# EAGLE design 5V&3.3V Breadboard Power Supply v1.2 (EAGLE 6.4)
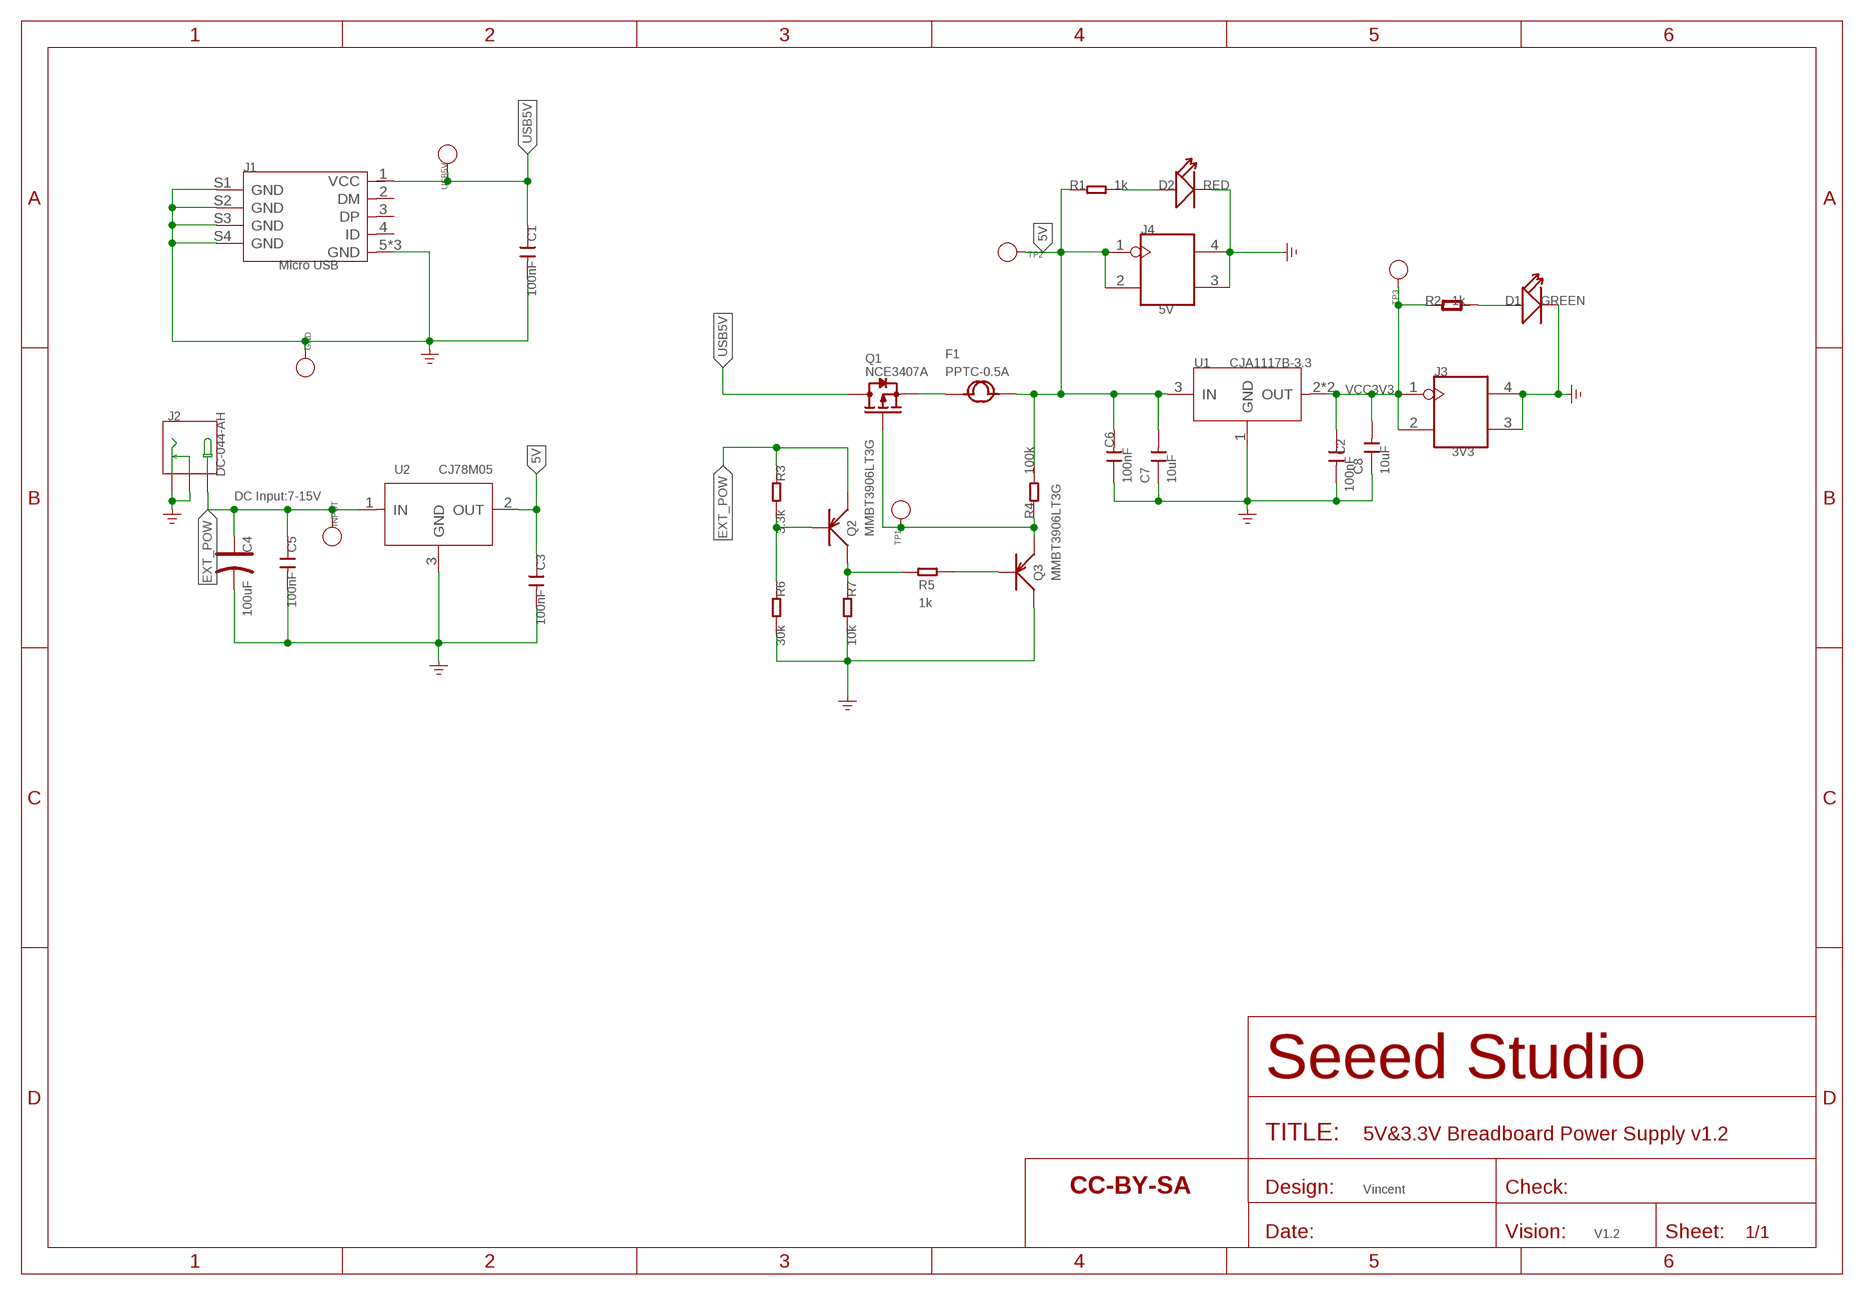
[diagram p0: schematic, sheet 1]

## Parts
C1  100nF  CAP-0603  [C0603]
C2  100nF  CAP-0603  [C0603]
C3  100nF  CAP-0603  [C0603]
C4  100uF  CAP_ELECTRO_D  [ELECTRO-SMD-D]
C5  100nF  CAP-0603  [C0603]
C6  100nF  CAP-0603  [C0603]
C7  10uF  CAP-0805  [C0805]
C8  10uF  CAP-0805  [C0805]
D1  GREEN  LED-0603  [LED-0603]
D2  RED  LED-0603  [D0603]
F1  PPTC-0.5A  FUSE'1206'  [F1206]
GND  DNP  PAD-TEST-POINT'4545'  [TP_4545]
INPUT  DNP  PAD-TEST-POINT'4545'  [TP_4545]
J1  Micro USB  USB-MICRO-5P'5+4P'  [5+4P-SMD-0.65-B]
J2  DC-044-AH  POWER-JACK-DC'DC-044'  [3P-L11.6*W9.6*H7.0MM]
J3  3V3  HEADER-2X2P-2.54  [2X2P-2.54-65/35MIL]
J4  5V  HEADER-2X2P-2.54  [2X2P-2.54-65/35MIL]
Q1  NCE3407A  MOSFET-P'SI2323CDS/SI2305DS<BR>'  [SOT23]
Q2  MMBT3906LT3G  TRANSISTOR-PNP-SOT23  [SOT23]
Q3  MMBT3906LT3G  TRANSISTOR-PNP-SOT23  [SOT23]
R1  1k  R-0603  [R0603]
R2  1k  R-0603  [R0603]
R3  3.3k  R-0603  [R0603]
R4  100k  R-0603  [R0603]
R5  1k  R-0603  [R0603]
R6  30k  R-0603  [R0603]
R7  10k  R-0603  [R0603]
TP1  DNP  PAD-TEST-POINT'4545'  [TP_4545]
TP2  DNP  PAD-TEST-POINT'4545'  [TP_4545]
TP3  DNP  PAD-TEST-POINT'4545'  [TP_4545]
U1  CJA1117B-3.3  PMIC-CJ1117'SOT89'  [SOT-89]
U2  CJ78M05  PMIC-CJ78M05CJ  [TO-252]
U$3  SEEEDSTUDIO-OPEN-SCH-FRAME  [SEEEDSTUDIO-PCB-FRAME]
USB5V  DNP  PAD-TEST-POINT'4545'  [TP_4545]

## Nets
5V: C3.1 C6.2 C7.2 F1.2 J4.1 J4.2 R1.1 R4.2 TP2.T U1.3(IN) U2.2(OUT)
EXT_POW: C4.+ C5.1 INPUT.T J2.+ Q2.2(E) R3.1 U2.1(IN)
EXT_PWR_SIG: Q1.1(G) Q3.2(E) R4.1 TP1.T
GND: C1.2 C2.2 C3.2 C4.- C5.2 C6.1 C7.1 C8.1 D1.- D2.- GND.T J1.5(GND) J1.S1(GND) J1.S2(GND) J1.S3(GND) J1.S4(GND) J1.S5(GND) J1.S6(GND) J2.- J2.CDN J3.3 J3.4 J4.3 J4.4 Q3.3(C) R6.2 R7.2 U1.1(GND) U2.3(GND) ; supply symbol labelled GND_POWER
N$1: D1.+ R2.2
N$2: Q2.1(B) R3.2 R6.1
N$3: D2.+ R1.2
N$8: Q3.1(B) R5.2
N$9: Q2.3(C) R5.1 R7.1
P5V [usbvcc]: F1.1 Q1.2(S)
USB5V: C1.1 J1.1(VCC) Q1.3(D) USB5V.T
VCC3V3: C2.1 C8.2 J3.1 J3.2 R2.1 TP3.T U1.2(OUT) U1.4(OUT)
Unconnected: J1.2(DM) J1.3(DP) J1.4(ID)

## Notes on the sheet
- DC Input:7-15V
- Vincent
- V1.2

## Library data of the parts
C1-C3 C5-C8 = OPL:CAP: Ceramic Capacitors
C4 = Discrete:CAP*: Electrolytic Capacitors,Tantalum Capacitors and Super Capacitors
D1 = OPL:LED
D2 = Discrete:LED*
F1 = Discrete:FUSE
GND INPUT TP1-TP3 USB5V = Discrete:PAD-TEST-POINT; PARTNO: DNP
J1 = Connector-new:USB-MICRO-5P: 5+4P-SMD-0.65-B:320010000;5+2P-SMD-0.65-AB:340032001
J2 = Connector-new:POWER-JACK-DC: 3P-L11.6*W9.6*H7.0MM:320120002;3P-L14.2*W11.0*H9.0MM:320120003
J3 J4 = Connector-new:HEADER-2X2P
Q1 = Discrete:MOSFET-P
Q2 Q3 = Discrete:TRANSISTOR-PNP*: PNP audion
R1 R3-R7 = Discrete:R*
R2 = OPL:R*
U1 = IC-new:PMIC-CJ*1117: Low Drop Fixed And Adjustable Positive Voltage Regulators http://www.datasheetcatalog.org/datasheet/SGSThomsonMicroelectronics/mXuqtqv.pdf
U2 = IC-new:PMIC-CJ78M05: 310030100
U$3 = moudle-new:SEEEDSTUDIO-OPEN-SCH-FRAME

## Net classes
0 default: width 0.152 mm, clearance 0.152 mm
3 usbvcc: width 0.152 mm, drill 0.152 mm, clearance 0.152 mm

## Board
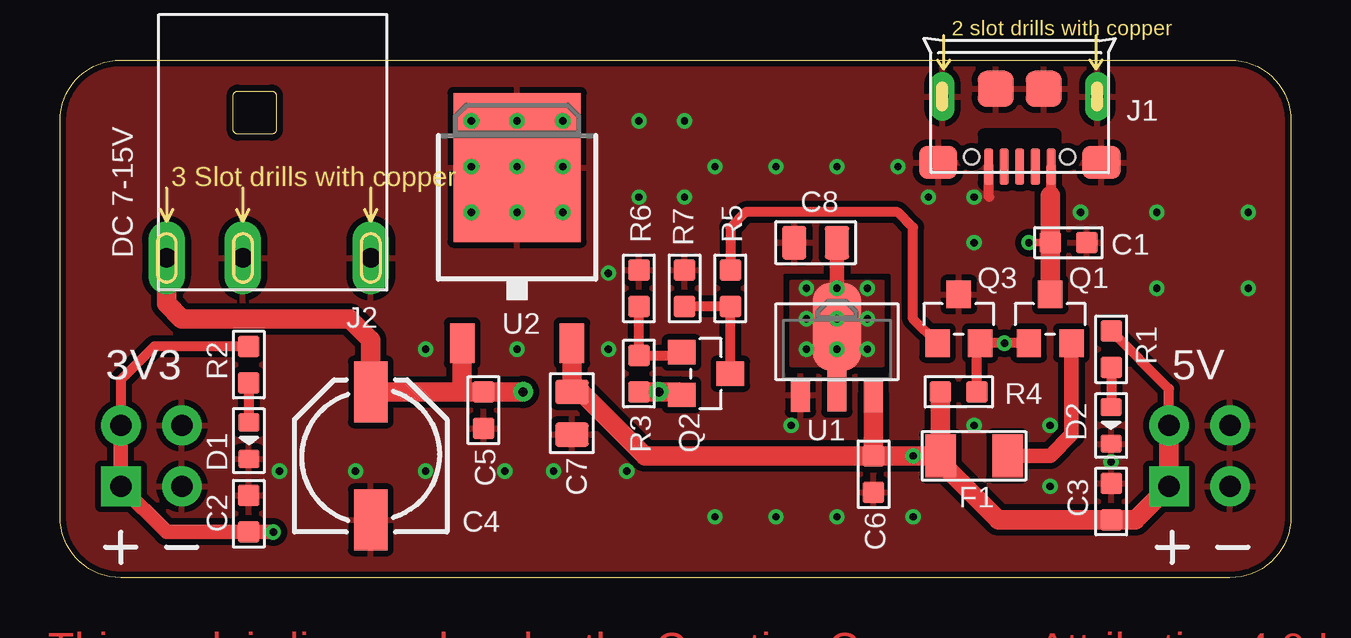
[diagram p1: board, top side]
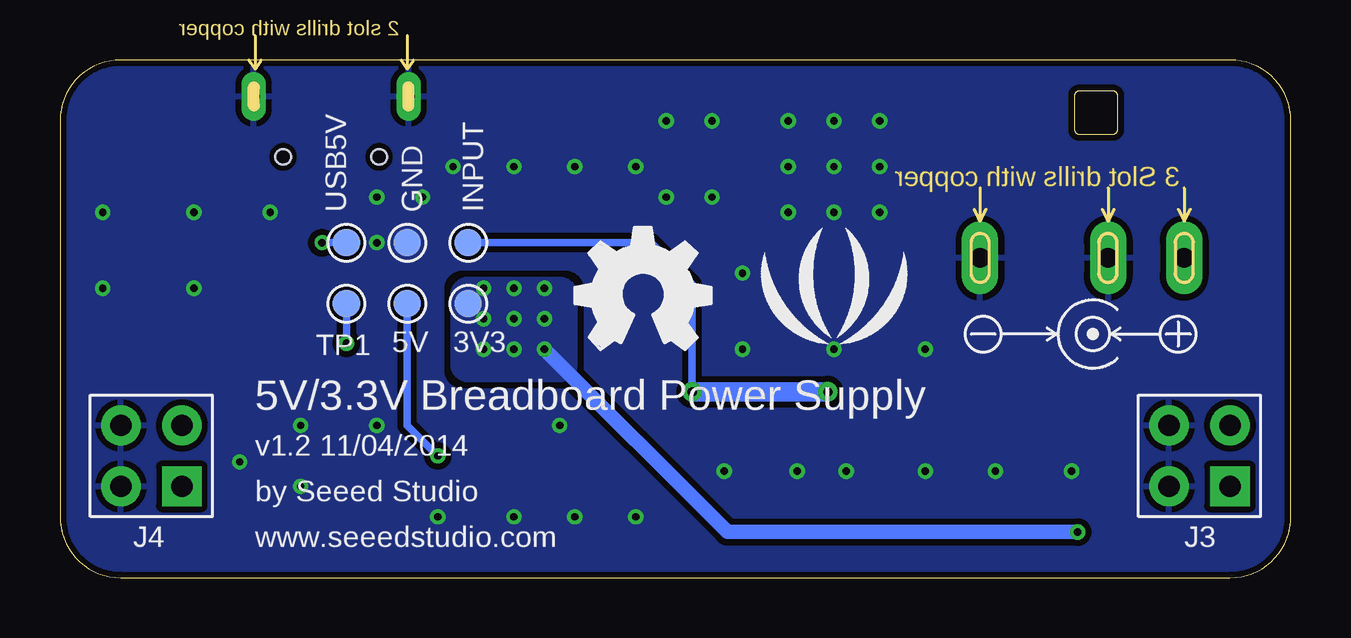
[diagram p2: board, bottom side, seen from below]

Size 51.31 x 21.59 mm. Coordinates in mm from the lower left corner, seen from the top.
Outline: 2.54,0 arc-90 0,2.54 0,19.05 arc-90 2.54,21.59 48.77,21.59 arc-90 51.31,19.05 51.31,2.54 arc-90 48.77,0 2.54,0
Copper layers (1*16): Top 0.035mm / dielectric 1.5mm / Bottom 0.035mm
Design rules "default": minimum track width 6mil, minimum drill 12mil, track to track 6mil, track to pad 6mil, pad to pad 6mil, via to via 6mil, smd to smd 0mil, copper to edge 10mil, drill to drill 10mil, minimum pad ring 10mil, minimum via ring 6mil, stop-mask expansion 2mil, vias tented up to drill 100mil, thermal gap 10mil

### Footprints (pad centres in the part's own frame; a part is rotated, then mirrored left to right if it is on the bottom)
C0603 = smd 0.889 x 0.889: 1 -0.762,0; 2 0.762,0
ELECTRO-SMD-D = smd 2.54 x 1.397: + 2.667,0; - -2.667,0
C0805 = smd 1.016 x 1.397: 1 -0.889,0; 2 0.889,0
LED-0603 = smd 0.762 x 0.889: + -0.762,0; - 0.762,0
D0603 = smd 0.762 x 0.889: + -0.762,0; - 0.762,0
F1206 = smd 1.27 x 1.778: 1 -1.397,0; 2 1.397,0
TP_4545 = smd 1.143 x 1.143: T 0,0
5+4P-SMD-0.65-B = smd 0.381 x 1.524: 1 -1.3,-0.25; 2 -0.65,-0.25; 3 0,-0.25; 4 0.65,-0.25; 5 1.3,-0.25 | smd 1.6 x 1.397: S1 -3.4,-0.427; S6 3.4,-0.427 | drill 0.508 pad 1.016 long: S2 -3.226,-3.175; S5 3.226,-3.175 | smd 1.5 x 1.5: S3 -1,-3.5; S4 1,-3.5 | hole 0.635: -2,-0.65; 2,-0.65
3P-L11.6*W9.6*H7.0MM = drill 0.813 pad 1.524 long: + 3.175,10.16; - -5.334,10.16; CDN 0,10.16
2X2P-2.54-65/35MIL = drill 0.889 pad 1.651 square: 1 -1.27,1.27 | drill 0.889 pad 1.651: 2 -1.27,-1.27; 3 1.27,-1.27; 4 1.27,1.27
SOT23 = smd 1.016 x 1.143: 1 -0.889,-1.016; 2 0.889,-1.016; 3 0,1.016
R0603 = smd 0.889 x 0.889: 1 -0.762,0; 2 0.762,0
SOT-89 = smd 0.8 x 1.4: 1 -1.524,-1.905; 3 1.524,-1.905 | smd 0.8 x 1.9: 2 0,-1.651 | smd 2.032 x 3.65: 4 0,0.94
TO-252 = smd 1.016 x 1.651: 1 -2.286,-4.826; 2 2.286,-4.826 | smd 5.3 x 6.2: 3 0,2.5

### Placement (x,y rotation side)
C1  42.04,13.97 0 top
C2  7.87,2.67 90 top
C3  43.81,3.17 90 top
C4  12.95,5.08 90 top
C5  17.65,6.98 270 top
C6  33.91,4.32 90 top
C7  21.34,6.86 90 top
C8  31.5,13.97 0 top
D1  7.87,5.71 270 top
D2  43.81,6.35 270 top
F1  38.1,5.08 180 top
GND  36.83,13.97 0 bottom
INPUT  34.29,13.97 0 bottom
J1  40.01,16.89 180 top
J2  7.62,23.5 180 top
J3  3.81,5.08 180 bottom
J4  47.5,5.08 180 bottom
Q1  41.27,10.79 0 top
Q2  26.92,8.51 270 top
Q3  37.47,10.79 0 top
R1  43.81,9.53 270 top
R2  7.87,8.89 270 top
R3  24.13,8.51 90 top
R4  37.47,7.75 180 top
R5  27.94,12.06 90 top
R6  24.13,12.06 90 top
R7  26.04,12.06 90 top
TP1  39.37,11.43 0 bottom
TP2  36.83,11.43 90 bottom
TP3  34.29,11.43 0 bottom
U1  32.38,9.53 0 top
U2  19.05,14.61 0 top
U$1  [LOGO_SILK]  19.05,11.43 0 bottom
U$2  [OSHW_FILLX200_NOTEXT]  29.84,9.53 0 bottom
U$3  not placed on the board
USB5V  39.37,13.97 0 bottom

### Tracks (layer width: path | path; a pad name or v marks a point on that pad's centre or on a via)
5V  (via drill 0.3 pad 0.64)
  Top 0.406: J4.2 46.23,7.87 R1.1
  Top 0.813: F1.2 R4.2 | U1.3 C6.2 | C6.2 v35.56,5.08 36.45,5.08 | 36.45,5.08 F1.2 | J4.2 J4.1 44.83,2.41 C3.1 39.12,2.41 36.45,5.08 | U2.2 C7.2 21.72,7.75 24.38,5.08 C6.2 | 36.7,4.83 F1.2
  Bottom 0.305: TP2.T 36.83,6.35 v35.56,5.08
EXT_POW  (via drill 0.38 pad 0.81)
  Top 0.61: 25.9,7.61 Q2.2
  Top 0.813: Q2.2 25.78,7.75 v24.96,7.75 R3.1 | J2.+ 4.45,11.43 5.08,10.79 12.06,10.79 12.95,9.91 C4.+ 16.76,7.75 | 16.76,7.75 C5.1 v19.3,7.75 | U2.1 16.76,7.75
  Bottom 0.305: INPUT.T 26.67,13.97 24.96,12.25 v24.96,7.75
  Bottom 0.813: v19.3,7.75 v24.96,7.75
EXT_PWR_SIG  (via drill 0.3 pad 0.64)
  Top 0.406: 38.48,9.78 v39.37,9.78 Q1.1 | 38.48,9.78 Q3.2 | R4.1 38.23,9.53 38.48,9.78
  Bottom 0.305: TP1.T v39.37,9.78
GND  (via drill 0.3 pad 0.64)
  Top 0.406: J1.5 38.7,15.9 38.73,15.88
  other vias: 17.14,19.05 19.05,19.05 20.95,19.05 17.14,17.15 17.14,15.24 20.95,15.24 20.95,17.15 19.05,17.15 19.05,15.24 9.14,4.45 12.32,4.45 15.24,4.45 22.86,12.7 18.54,4.45 20.57,4.45 23.62,4.45 30.48,6.35 29.84,2.54 32.38,2.54 35.56,2.54 27.3,2.54 36.2,15.88 41.27,6.35 38.1,6.35 42.55,15.24 45.72,15.24 45.72,12.06 49.53,12.06 49.53,15.24 38.1,13.97 38.1,15.88 15.24,9.53 22.86,9.53 24.13,15.88 26.04,15.88 24.13,19.05 26.04,19.05 27.3,17.15 29.84,17.15 32.38,17.15 34.92,17.15 43.81,4.83 41.27,3.81 19.05,9.53
  pour Bottom (isolate 0.254, rank 2): 0,21.59 51.44,21.59 51.44,0 0,0
  pour Top (isolate 0.254, rank 2): 0,21.59 51.44,21.59 51.44,0 0,0
N$1
  Top 0.406: R2.2 D1.+
N$2
  Top 0.406: R6.1 R3.2 25.78,9.27 Q2.1
N$3
  Top 0.406: R1.2 D2.+
N$8
  Top 0.406: Q3.1 35.56,10.79 35.56,14.61 34.92,15.24 28.57,15.24 27.94,14.61 R5.2
N$9
  Top 0.406: Q2.3 R5.1 R7.1
P5V
  Top 0.61: Q1.2 42.16,5.97 41.27,5.08 F1.1
USB5V  (via drill 0.3 pad 0.64)
  Top 0.305: v40.39,13.97 C1.1
  Top 0.406: J1.1 41.3,15.9 41.27,15.88 41.27,15.94
  Top 0.813: 41.27,15.94 C1.1 Q1.3
  Bottom 0.305: USB5V.T v40.39,13.97
VCC3V3  (via drill 0.3 pad 0.64)
  Top 0.305: U1.2 v32.38,9.53
  Top 0.406: R2.1 3.94,9.65 2.54,8.26 J3.2
  Top 0.61: C8.2 v32.38,12.06 | v8.89,1.91 C2.1 4.45,1.91 J3.1 J3.2
  Bottom 0.61: v31.11,9.53 23.5,1.91 v8.89,1.91
  other vias: 33.66,9.53 32.38,10.79 31.11,10.79 33.66,10.79 33.66,12.06 31.11,12.06
  pour Top (isolate 0.254, no thermals): 30.48,8.89 34.29,8.89 34.29,12.32 30.48,12.32
  pour Bottom (isolate 0.254, no thermals): 29.84,11.81 29.84,8.89 arc90 30.48,8.26 34.29,8.26 arc90 34.92,8.89 34.92,11.81 arc90 34.29,12.45 30.48,12.45 arc90

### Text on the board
tPlace: DC 7-15V | 3V3 | 5V | D2 | D1
bPlace: 3V3 | 5V | 5V/3.3V Breadboard Power Supply | v1.2 11/04/2014 | by Seeed Studio | www.seeedstudio.com
Reference: J8 | JST | MINIUSB | 1K | 1K | J1 | GREEN | GREEN | J6 | J2 | 10U | 10N | J7 | J3 | 10U | 100N | J5 | J4 | 100U

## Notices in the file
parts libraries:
moudle-new: This work is licensed under the Creative Commons Attribution 4.0 International License.
To view a copy of this license,visit:
http://creativecommons.org/licenses/by-sa/4.0
moudle-new: CC-BY-SA
